| TEXAS INSTRUMENTS INCORPORATED
| IBIS Model of SN74AVC4T245
| 4-BIT DUAL-SUPPLY BUS TRANSCEIVER WITH CONFIGURABLE VOLTAGE
| TRANSLATION AND 3-STATE OUPUTS
| This file contains package information for the following:
|  SOIC 16-pin (D) package as [Component] AVC4T245_D
|  QFN 16-pin (RGY) package as [Component] AVC4T245_RGY
|  TSSOP 16-pin (PW) package as [Component] AVC4T245_PW
|  TVSOP 16-pin (DGV) package as [Component] AVC4T245_DGV
|  QFN 16-pin (RSV) package as [Component] AVC4T245_RSV
| This device can be powered at the following Vccs:
|  1.2 volt Vcc
|  1.5 volt Vcc
|  1.8 volt Vcc
|  2.5 volt Vcc
|  3.3 volt Vcc
| This file provides unique models under the [Model Selector] for each Vcc.
| For operation at a specific Vcc, select the appropriate model after each
| [Model Selector] keyword.
[IBIS Ver]   4.1
[Comment char]  |_char
[File Name]   sn74avc4t245.ibs
[File Rev]   1.3 | x_die
[Date]   April 8, 2014
[Source]   Data created from TI-SPICE simulations at TI-SLL.
   Texas Instruments Incorporated.
   Analog-eLab, HPA
   12500 TI Blvd
   Dallas, TX -75243
   For Support e-mail: elab_ibis@list.ti.com
[Notes]   Revision History
   Rev 1.3: 04/08/14
   - Correct Pin name assignments on RSV package
   Rev 1.2: 04/04/14
   - Add RSV package component
   Rev 1.1: 02/15/06
   - Power clamp data deleted as there is no power-clamp diode.
   - Due to the fact that the Device is 4.6-V Input/Output
   tolarent, the I/O models has some Non-Monotonic Warnings.
   Rev 1.0 Initial Release
[Disclaimer]  This model is designed as an aid for customers of Texas Instruments
 TI and its licensors and suppliers make no warranties, either expressed
 or implied, with respect to this  model, including the warranties of
 merchantability or fitness for a particular purpose.
 The model is provided solely on an "as is" basis. The entire risk as to
 its quality and performance is with the customer.
[Copyright] (C)Copyright 2014 Texas Instruments Incorporated.
   All rights reserved.
| Component AVC4T245_D 16-pin SOIC
[Component]   AVC4T245_D
[Manufacturer]   Texas Instruments, Inc.
[Package]
|   typ   min   max
R_pkg   3.900e-02   2.800e-02   4.900e-02
L_pkg   3.453e-09   2.350e-09   4.375e-09
C_pkg   5.210e-13   2.540e-13   7.080e-13
[Pin]   signal_name   model_name   R_pin   L_pin   C_pin
1   VCCA   POWER   4.200e-02   4.336e-09   7.030e-13
2   1DIR   AVC4T245_DIR   4.900e-02   3.778e-09   6.340e-13
3   2DIR   AVC4T245_DIR   2.800e-02   3.449e-09   5.180e-13
4   1A1   AVC4T245_IO   2.900e-02   2.393e-09   2.540e-13
5   1A2   AVC4T245_IO   2.800e-02   2.350e-09   2.640e-13
6   2A1   AVC4T245_IO   4.800e-02   3.312e-09   4.830e-13
7   2A2   AVC4T245_IO   4.300e-02   3.629e-09   6.040e-13
8   GND   GND   4.400e-02   4.375e-09   7.080e-13
9   GND   GND   4.200e-02   4.336e-09   7.030e-13
10   2B2   AVC4T245_IO   4.900e-02   3.778e-09   6.340e-13
11   2B1   AVC4T245_IO   2.800e-02   3.449e-09   5.180e-13
12   1B2   AVC4T245_IO   2.900e-02   2.393e-09   2.550e-13
13   1B1   AVC4T245_IO   2.800e-02   2.350e-09   2.640e-13
14   2NOE   AVC4T245_NOE   4.800e-02   3.312e-09   4.830e-13
15   1NOE   AVC4T245_NOE   4.300e-02   3.629e-09   6.040e-13
16   VCCB   POWER   4.400e-02   4.375e-09   7.080e-13
| Component AVC4T245_RGY 16-pin QFN
[Component]   AVC4T245_RGY
[Manufacturer]   Texas Instruments, Inc.
[Package]
|   typ   min   max
R_pkg   3.300e-02   2.900e-02   3.900e-02
L_pkg   7.470e-10   6.630e-10   8.830e-10
C_pkg   3.150e-13   3.030e-13   3.300e-13
[Pin]   signal_name   model_name   R_pin   L_pin   C_pin
1   VCCA   POWER   3.400e-02   7.740e-10   3.030e-13
2   1DIR   AVC4T245_DIR   3.400e-02   7.570e-10   3.110e-13
3   2DIR   AVC4T245_DIR   3.800e-02   8.510e-10   3.270e-13
4   1A1   AVC4T245_IO   2.900e-02   6.630e-10   3.110e-13
5   1A2   AVC4T245_IO   2.900e-02   6.640e-10   3.110e-13
6   2A1   AVC4T245_IO   3.000e-02   6.730e-10   3.110e-13
7   2A2   AVC4T245_IO   2.900e-02   6.650e-10   3.110e-13
8   GND   GND   3.300e-02   7.420e-10   3.170e-13
9   GND   GND   3.400e-02   7.640e-10   3.100e-13
10   2B2   AVC4T245_IO   3.200e-02   7.300e-10   3.140e-13
11   2B1   AVC4T245_IO   3.800e-02   8.590e-10   3.300e-13
12   1B2   AVC4T245_IO   3.600e-02   8.120e-10   3.220e-13
13   1B1   AVC4T245_IO   3.100e-02   7.050e-10   3.140e-13
14   2NOE   AVC4T245_NOE   3.200e-02   7.210e-10   3.150e-13
15   1NOE   AVC4T245_NOE   3.000e-02   6.840e-10   3.140e-13
16   VCCB   POWER   3.900e-02   8.830e-10   3.210e-13
| Component AVC4T245_PW 16-pin TSSOP
[Component]   AVC4T245_PW
[Manufacturer]   Texas Instruments, Inc.
[Package]
|   typ   min   max
R_pkg   4.500e-02   3.800e-02   5.100e-02
L_pkg   2.593e-09   2.447e-09   3.080e-09
C_pkg   2.810e-13   2.430e-13   3.770e-13
[Pin]   signal_name   model_name   R_pin   L_pin   C_pin
1   VCCA   POWER   4.000e-02   3.080e-09   3.770e-13
2   1DIR   AVC4T245_DIR   3.800e-02   2.458e-09   2.810e-13
3   2DIR   AVC4T245_DIR   5.100e-02   2.512e-09   2.550e-13
4   1A1   AVC4T245_IO   5.100e-02   2.447e-09   2.430e-13
5   1A2   AVC4T245_IO   5.100e-02   2.447e-09   2.430e-13
6   2A1   AVC4T245_IO   5.100e-02   2.512e-09   2.550e-13
7   2A2   AVC4T245_IO   3.800e-02   2.458e-09   2.810e-13
8   GND   GND   4.000e-02   3.080e-09   3.770e-13
9   GND   GND   3.900e-02   2.832e-09   3.160e-13
10   2B2   AVC4T245_IO   3.800e-02   2.460e-09   2.790e-13
11   2B1   AVC4T245_IO   5.100e-02   2.512e-09   2.550e-13
12   1B2   AVC4T245_IO   5.100e-02   2.447e-09   2.430e-13
13   1B1   AVC4T245_IO   5.100e-02   2.447e-09   2.430e-13
14   2NOE   AVC4T245_NOE   5.100e-02   2.512e-09   2.550e-13
15   1NOE   AVC4T245_NOE   3.800e-02   2.459e-09   2.790e-13
16   VCCB   POWER   3.900e-02   2.832e-09   3.160e-13
| Component AVC4T245_DGV 16-pin TVSOP
[Component]   AVC4T245_DGV
[Manufacturer]   Texas Instruments, Inc.
[Package]
|   typ   min   max
R_pkg   3.900e-02   3.300e-02   4.500e-02
L_pkg   2.543e-09   2.320e-09   2.938e-09
C_pkg   3.860e-13   3.340e-13   4.490e-13
[Pin]   signal_name   model_name   R_pin   L_pin   C_pin
1   VCCA   POWER   3.500e-02   2.907e-09   4.170e-13
2   1DIR   AVC4T245_DIR   4.200e-02   2.558e-09   4.460e-13
3   2DIR   AVC4T245_DIR   3.800e-02   2.341e-09   3.450e-13
4   1A1   AVC4T245_IO   3.800e-02   2.320e-09   3.340e-13
5   1A2   AVC4T245_IO   3.900e-02   2.322e-09   3.340e-13
6   2A1   AVC4T245_IO   3.800e-02   2.353e-09   3.420e-13
7   2A2   AVC4T245_IO   4.000e-02   2.536e-09   4.410e-13
8   GND   GND   3.300e-02   2.897e-09   4.180e-13
9   GND   GND   3.500e-02   2.927e-09   4.190e-13
10   2B2   AVC4T245_IO   4.500e-02   2.632e-09   4.490e-13
11   2B1   AVC4T245_IO   3.900e-02   2.368e-09   3.470e-13
12   1B2   AVC4T245_IO   3.900e-02   2.330e-09   3.350e-13
13   1B1   AVC4T245_IO   3.900e-02   2.320e-09   3.350e-13
14   2NOE   AVC4T245_NOE   3.900e-02   2.361e-09   3.450e-13
15   1NOE   AVC4T245_NOE   4.100e-02   2.573e-09   4.460e-13
16   VCCB   POWER   3.500e-02   2.938e-09   4.200e-13
| Component AVC4T245_RSV 16-pin QFN
[Component]   AVC4T245_RSV
[Manufacturer]   Texas Instruments, Inc.
[Package]   |16 pin QFN RSV
|   typ   min   max
R_pkg   0.0937   0.0686   0.1241
L_pkg   0.5757n   0.3926n   0.7965n
C_pkg   0.0726p   0.0692p   0.0773p
[Pin]   signal_name   model_name   R_pin   L_pin   C_pin
1   1NOE   AVC4T245_NOE   0.07703   0.45677n   0.07178p
2   VCCB   POWER   0.06898   0.40049n   0.06997p
3   VCCA   POWER   0.06869   0.39847n   0.07026p
4   1DIR   AVC4T245_DIR   0.08221   0.49360n   0.07444p
5   2DIR   AVC4T245_DIR   0.10720   0.67397n   0.07058p
6   1A1   AVC4T245_IO   0.10723   0.67312n   0.07251p
7   1A2   AVC4T245_IO   0.11302   0.71510n   0.07465p
8   2A1   AVC4T245_IO   0.12407   0.79611n   0.07713p
9   2A2   AVC4T245_IO   0.08071   0.47831n   0.07266p
10   GND   GND   0.06855   0.39255n   0.06920p
11   GND   GND   0.06882   0.39450n   0.06934p
12   2B2   AVC4T245_IO   0.08072   0.47837n   0.07268p
13   2B1   AVC4T245_IO   0.12412   0.79653n   0.07727p
14   1B2   AVC4T245_IO   0.11308   0.71557n   0.07484p
15   1B1   AVC4T245_IO   0.10730   0.67361n   0.07273p
16   2NOE   AVC4T245_NOE   0.10725   0.67435n   0.07092p
| Model AVC4T245_NOE
[Model Selector]   AVC4T245_NOE
AVC4T245_NOE_12   1.2 volt Vcc
AVC4T245_NOE_15A   1.5 volt Vcc
AVC4T245_NOE_18   1.8 volt Vcc
AVC4T245_NOE_25   2.5 volt Vcc
AVC4T245_NOE_33   3.3 volt Vcc
| Model AVC4T245_DIR
[Model Selector]   AVC4T245_DIR
AVC4T245_DIR_12   1.2 volt Vcc
AVC4T245_DIR_15A   1.5 volt Vcc
AVC4T245_DIR_18   1.8 volt Vcc
AVC4T245_DIR_25   2.5 volt Vcc
AVC4T245_DIR_33   3.3 volt Vcc
| Model AVC4T245_IO
[Model Selector]   AVC4T245_IO
AVC4T245_IO_12   1.2 volt Vcc
AVC4T245_IO_15A   1.5 volt Vcc
AVC4T245_IO_18   1.8 volt Vcc
AVC4T245_IO_25   2.5 volt Vcc
AVC4T245_IO_33   3.3 volt Vcc
| Models and submodels in the file (15): AVC4T245_NOE_12 (Input), AVC4T245_NOE_15A (Input), AVC4T245_NOE_18 (Input), AVC4T245_NOE_25 (Input), AVC4T245_NOE_33 (Input), AVC4T245_DIR_12 (Input), AVC4T245_DIR_15A (Input), AVC4T245_DIR_18 (Input), AVC4T245_DIR_25 (Input), AVC4T245_DIR_33 (Input), AVC4T245_IO_12 (I/O), AVC4T245_IO_15A (I/O), AVC4T245_IO_18 (I/O), AVC4T245_IO_25 (I/O), AVC4T245_IO_33 (I/O)
